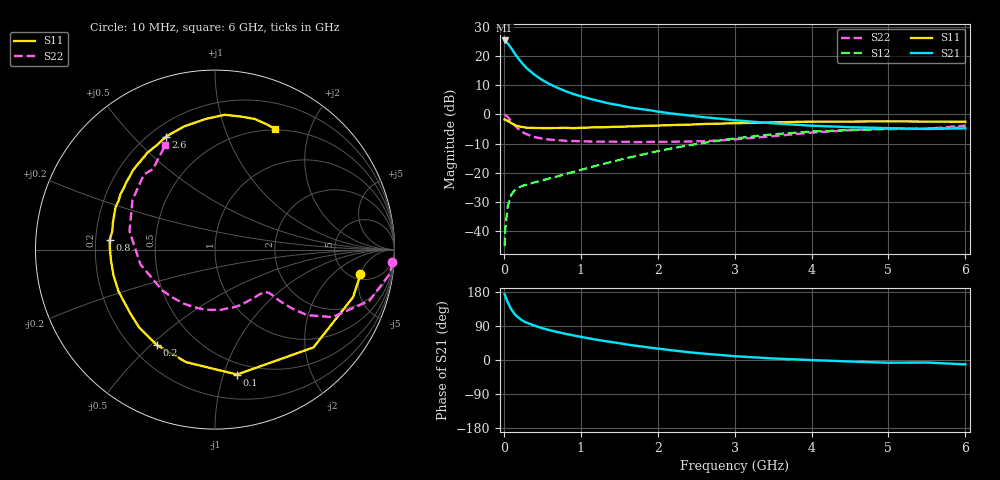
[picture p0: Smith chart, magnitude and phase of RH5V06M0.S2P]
! SIEMENS Small Signal Semiconductors
! BFR106
! Si NPN RF Bipolar Junction Transistor in SOT23
! VCE = 5 V  IC = 6 mA
! Common Emitter S-Parameters:  August  1996
# GHz  S  MA  R  50
!  f  S11  S21  S12  S22
! GHz  MAG  ANG  MAG  ANG  MAG  ANG  MAG  ANG
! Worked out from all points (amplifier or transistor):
!   36 points, 10 MHz to 6 GHz, reference 50 ohm
!   highest |S21| = 25.5 dB at 10 MHz (marker M1)
!   |S21| within 3 dB of that: start of sweep to 104.7 MHz
!   unconditionally stable (mu >= 1): 587.5 MHz to 1.874 GHz; 5.01 GHz to end of sweep
!   at 250 MHz: K = 0.56, MSG = 20.9 dB, |S12| = -24.5 dB
!   at 1.4 GHz: K = 1.12, MAG = 7.9 dB, |S12| = -16.3 dB
!   at 6 GHz: K = 1.01, MAG = -0.9 dB, |S12| = -4.5 dB
!   S11 on the Smith chart (normalised r, x): 10 MHz: 5.88, -5.03; 100 MHz: 0.40, -1.11; 200 MHz: 0.30, -0.52; 800 MHz: 0.26, +0.04; 2.6 GHz: 0.26, +0.62; 6 GHz: 0.48, +1.50
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0.01  0.8223 -9.7  18.81 173.4  0.0054 88.3  0.9914 -4.1
0.02  0.8135 -19.0  18.5 168.2  0.0112 81.5  0.9824 -8.0
0.05  0.7732 -44.8  16.8 152.0  0.0259 68.3  0.9053 -18.4
0.1  0.7068 -80.0  13.62 132.7  0.0425 54.0  0.7547 -29.9
0.15  0.6475 -104.4  10.74 118.8  0.0509 46.3  0.6309 -35.4
0.2  0.6227 -121.4  8.801 110.2  0.0558 43.3  0.5498 -37.2
0.25  0.606 -134.1  7.313 103.0  0.0595 41.3  0.489 -38.1
0.3  0.5909 -142.9  6.228 98.3  0.0622 41.6  0.4547 -38.5
0.4  0.5859 -156.5  4.823 90.5  0.0679 43.2  0.4081 -38.4
0.5  0.5835 -165.9  3.909 83.9  0.0734 45.8  0.3826 -38.8
0.6  0.5827 -174.0  3.306 78.5  0.0796 48.8  0.3692 -40.2
0.8  0.5894 174.9  2.523 69.2  0.0941 53.9  0.3528 -44.4
1.1  0.5955 160.2  1.892 57.4  0.1205 59.7  0.3436 -53.2
1.3  0.6023 153.0  1.626 50.4  0.1419 61.8  0.3397 -59.9
1.6  0.6208 142.6  1.349 41.0  0.1775 63.1  0.3381 -71.6
2.2  0.6583 124.8  1.032 25.2  0.2632 59.7  0.3394 -99.0
2.6  0.6859 113.4  0.897 16.8  0.3247 54.5  0.348 -120.4
3.5  0.7303 93.9  0.704 4.0  0.4565 38.6  0.4238 -168.9
4.5  0.7552 78.9  0.604 -4.0  0.5401 19.2  0.5368 148.9
5  0.7609 73.0  0.582 -7.2  0.5604 11.1  0.5764 133.4
5.5  0.7548 67.6  0.563 -6.7  0.5696 6.9  0.5659 127.7
6  0.7514 63.8  0.578 -11.5  0.5986 -1.2  0.6444 115.5
